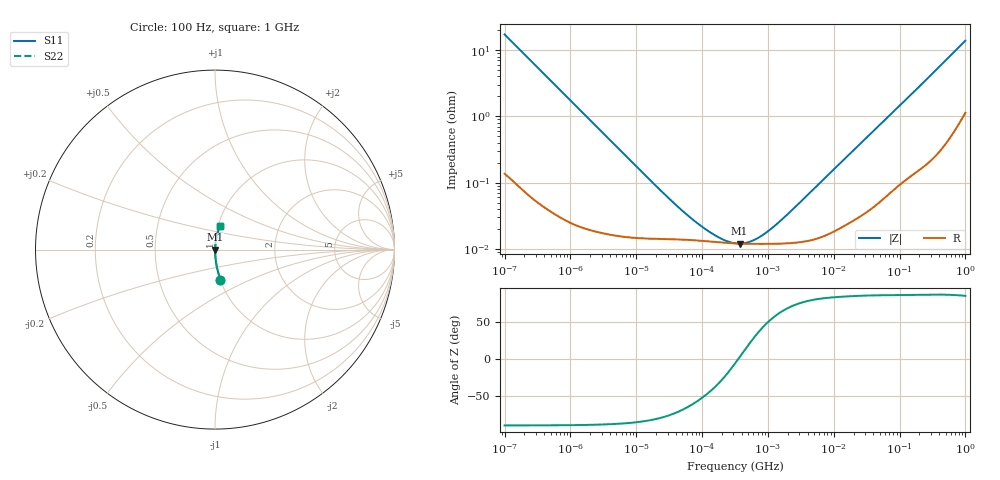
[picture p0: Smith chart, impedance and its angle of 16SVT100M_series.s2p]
!  *** S-Parameter ***
!  Copyright (C) Panasonic Industry
!  Conductive Polymer Aluminum Soild Capacitor (OS-CON)
!  Parts No. 16SVT100M
!  Connection Mode : Series
!  1  o---||---o  2
!  GND o--------o GND
!  Conditions : Temperature = 20 degC  DC Bias = 0 V
! Frequency Range : 100Hz  -  1GHz  [ 401 Steps ]
# Hz S RI R 50
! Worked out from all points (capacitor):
!   401 points, 100 Hz to 1 GHz, reference 50 ohm
!   read as one part in series: C = 92.3 uF near 108.4 Hz
!   lowest |Z| = 12 mohm at 371.5 kHz (marker M1)
!   series resonance near 354 kHz, so ESL is about 2.2 nH
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100  0.03 -0.1668  0.97 0.1668  0.97 0.1668  0.03 -0.1668
108.3927  0.0258 -0.1546  0.9742 0.1546  0.9742 0.1546  0.0258 -0.1546
175.7924  0.0104 -0.0972  0.9896 0.0972  0.9896 0.0972  0.0104 -0.0972
309.0295  0.00363 -0.0558  0.9964 0.0558  0.9964 0.0558  0.00363 -0.0558
1487.647  0.000347 -0.0117  0.9997 0.0117  0.9997 0.0117  0.000347 -0.0117
22130.95  0.000142 -0.000793  0.9999 0.000793  0.9999 0.000793  0.000142 -0.000793
53703.18  0.000138 -0.000327  0.9999 0.000327  0.9999 0.000327  0.000138 -0.000327
106536.9  0.000131 -0.000159  0.9999 0.000159  0.9999 0.000159  0.000131 -0.000159
194984.5  0.000125 -6.93e-05  0.9999 6.93e-05  0.9999 6.93e-05  0.000125 -6.93e-05
248313.3  0.000123 -4.02e-05  0.9999 4.02e-05  0.9999 4.02e-05  0.000123 -4.02e-05
316227.8  0.000121 -1.27e-05  0.9999 1.27e-05  0.9999 1.27e-05  0.000121 -1.27e-05
371535.2  0.00012 5.45e-06  0.9999 -5.45e-06  0.9999 -5.45e-06  0.00012 5.45e-06
454464.5  0.000119 2.85e-05  0.9999 -2.85e-05  0.9999 -2.85e-05  0.000119 2.85e-05
578762  0.000119 5.8e-05  0.9999 -5.8e-05  0.9999 -5.8e-05  0.000119 5.8e-05
938642  0.000119 0.000129  0.9999 -0.000129  0.9999 -0.000129  0.000119 0.000129
1717908  0.00012 0.000265  0.9999 -0.000265  0.9999 -0.000265  0.00012 0.000265
4704354  0.000137 0.000748  0.9999 -0.000748  0.9999 -0.000748  0.000137 0.000748
6.99842e7  0.000786 0.0103  0.9992 -0.0103  0.9992 -0.0103  0.000786 0.0103
3.368992e8  0.00461 0.0468  0.9954 -0.0468  0.9954 -0.0468  0.00461 0.0468
5.688529e8  0.0107 0.078  0.9893 -0.078  0.9893 -0.078  0.0107 0.078
9.225714e8  0.0254 0.1235  0.9746 -0.1235  0.9746 -0.1235  0.0254 0.1235
1e9  0.0294 0.1329  0.9706 -0.1329  0.9706 -0.1329  0.0294 0.1329
